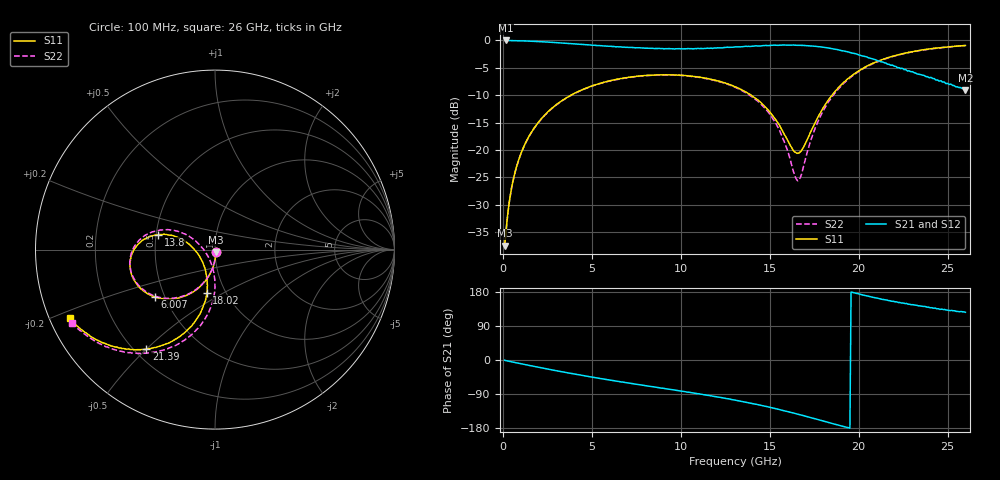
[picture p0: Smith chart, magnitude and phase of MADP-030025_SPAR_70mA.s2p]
!Mean
# HZ S DB R 50
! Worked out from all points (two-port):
!   400 points, 100 MHz to 26 GHz, reference 50 ohm
!   highest |S21| = -0.03 dB at 164.9 MHz (marker M1); lowest = -9.1 dB at 26 GHz (marker M2)
!   |S21| within 3 dB of the highest: start of sweep to 20.45 GHz
!   lowest |S11| = -37.4 dB at 100 MHz (marker M3), VSWR 1.03, Z = 50.4 - j1.29 ohm
!   |S11| at or under -10 dB: start of sweep to 3.832 GHz; 13.95 GHz to 18.5 GHz (4.546 GHz wide, 28 % of centre)
!   |S22| runs from -37.5 to -0.9 dB; largest |S21 - S12| = 0.0058
!   S11 on the Smith chart (normalised r, x): 100 MHz: 1.01, -0.03; 6.007 GHz: 0.44, -0.28; 13.8 GHz: 0.51, +0.10; 18.02 GHz: 0.82, -0.42; 21.39 GHz: 0.25, -0.50; 26 GHz: 0.06, -0.22
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1e8  -37.42 -72.0  -0.04 -0.8  -0.03 -0.8  -37.52 -72.7
1.6491e8  -35.39 -76.8  -0.03 -1.6  -0.04 -1.5  -35.30 -77.3
3.5965e8  -29.55 -84.5  -0.05 -3.5  -0.05 -3.5  -29.58 -84.6
5.5439e8  -25.86 -88.8  -0.06 -5.4  -0.07 -5.4  -25.94 -88.6
1.3333e9  -18.32 -99.6  -0.13 -12.9  -0.13 -12.9  -18.37 -99.7
2.6316e9  -12.75 -113.0  -0.34 -24.9  -0.34 -24.9  -12.79 -113.3
4.4491e9  -9.02 -129.4  -0.75 -40.6  -0.75 -40.6  -9.05 -130.0
6.007e9  -7.39 -142.1  -1.09 -53.0  -1.10 -52.9  -7.41 -142.9
8.7982e9  -6.30 -162.3  -1.47 -73.3  -1.48 -73.3  -6.33 -163.7
1.1005e10  -6.68 -177.1  -1.48 -89.0  -1.48 -89.1  -6.73 -179.4
1.3082e10  -8.51 169.2  -1.20 -106.2  -1.22 -106.2  -8.59 165.3
1.3796e10  -9.67 165.3  -1.09 -112.6  -1.11 -112.7  -9.82 160.2
1.5419e10  -14.85 163.6  -0.89 -129.2  -0.89 -129.3  -15.57 152.6
1.6588e10  -20.59 -149.1  -0.92 -143.0  -0.92 -143.1  -25.61 -149.8
1.6782e10  -20.13 -134.0  -0.92 -145.4  -0.92 -145.3  -24.50 -122.1
1.7367e10  -16.27 -107.8  -1.03 -152.7  -1.03 -152.6  -17.70 -92.8
1.8016e10  -12.26 -100.7  -1.26 -161.1  -1.27 -161.1  -12.80 -90.3
1.9379e10  -7.02 -107.0  -2.09 -178.1  -2.08 -178.1  -7.18 -101.2
2.1391e10  -3.43 -124.6  -4.00 159.8  -3.98 160.0  -3.50 -121.1
2.1716e10  -3.10 -127.2  -4.37 156.6  -4.37 156.5  -3.15 -124.0
2.4053e10  -1.54 -143.9  -6.76 137.8  -6.73 138.3  -1.56 -141.8
2.6e10  -0.95 -154.7  -9.08 125.9  -8.95 125.9  -0.95 -153.0
